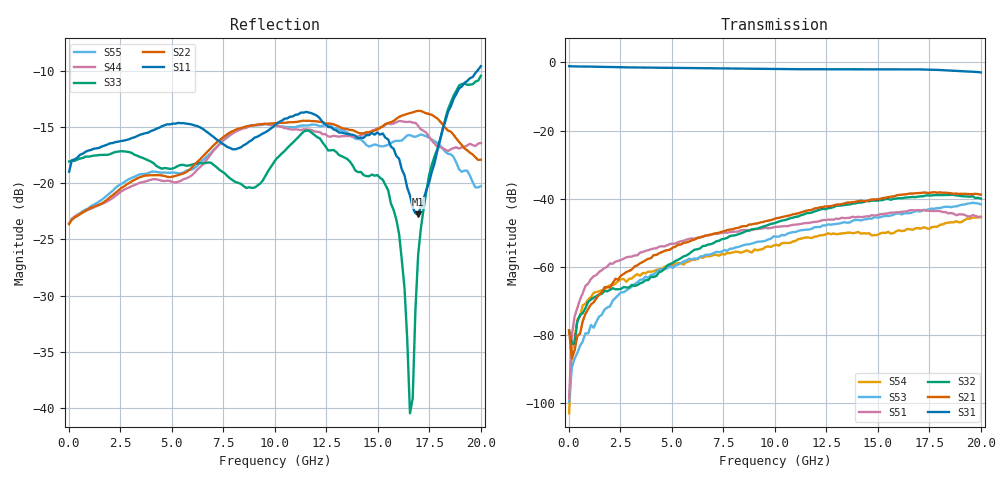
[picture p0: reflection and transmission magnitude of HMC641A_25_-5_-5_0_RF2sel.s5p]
! Device:  HMC641A
! Description: GaAs MMIC SP4T NON-REFLECTIVE
! Frequency:  0.01 -  18 GHz
! Ports:
! RFC = Port 1
! RF1 = Port 2
! RF2 = Port 3
! RF3 = Port 4
! RF4 = Port 5
! State: RF2 selected
! Vss:  -5 Volts
! Control A  -5 Volts
! Control B:  0 Volts
! Temperature = +25 C
! Data: Data was collected using a calibrated network analyzer.
!  The reference plane is the edge of the device.
! Note: Analog Devices supplies this data as a sample of measured data for this product.
!  Your particular data for this product may vary.
!  Analog Devices reserves the right to change this data at anytime
# Hz S DB R 50.0
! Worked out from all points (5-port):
!   152 points, 10 MHz to 20.01 GHz, reference 50 ohm
!   strongest paths, dB at 10 MHz, 5.043 GHz, 10.08 GHz, 15.11 GHz, 20.01 GHz:
!     S31: -1.1, -1.6, -1.9, -2.1, -3.0
!     S21: -78.6, -54.4, -45.7, -40.0, -38.8
!     S32: -78.7, -58.8, -47.0, -40.4, -40.0
!     S51: -98.6, -53.2, -48.2, -44.6, -45.4
!     S53: -99.6, -60.3, -51.1, -45.4, -41.6
!     S54: -102.9, -59.5, -53.5, -50.2, -45.2
!   lowest |S11| = -22.8 dB at 16.96 GHz (marker M1), VSWR 1.16, Z = 43.4 - j1.75 ohm
!   |S11| at or under -10 dB: start of sweep to 19.85 GHz
